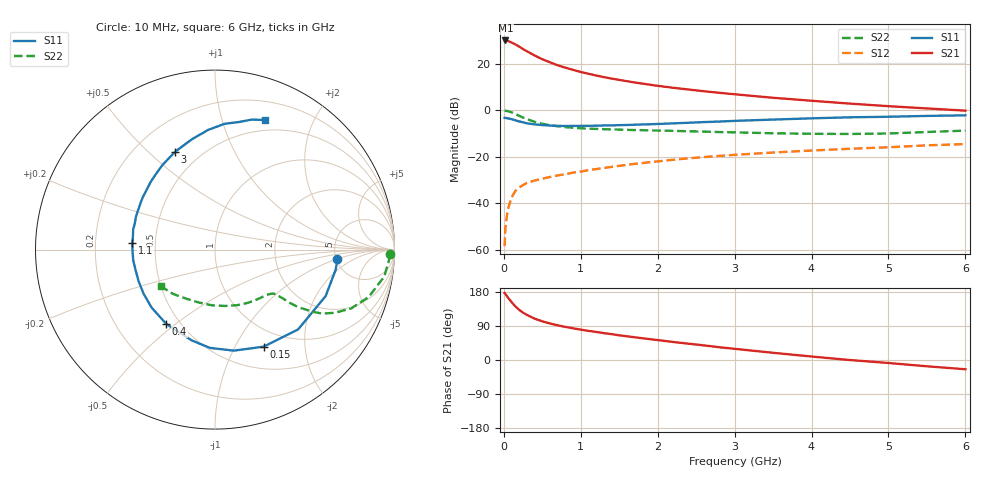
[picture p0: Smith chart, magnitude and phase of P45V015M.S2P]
! SIEMENS Small Signal Semiconductors
! BFP182
! Si NPN RF Bipolar Junction Transistor in SOT143
! VCE = 5 V  IC = 15 mA
! Common Emitter S-Parameters:  March  1996
# GHz  S  MA  R  50
!  f  S11  S21  S12  S22
! GHz  MAG  ANG  MAG  ANG  MAG  ANG  MAG  ANG
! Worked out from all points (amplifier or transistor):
!   36 points, 10 MHz to 6 GHz, reference 50 ohm
!   highest |S21| = 29.9 dB at 20 MHz (marker M1)
!   |S21| within 3 dB of that: start of sweep to 216.3 MHz
!   unconditionally stable (mu >= 1): 978.4 MHz to 5.403 GHz
!   at 250 MHz: K = 0.40, MSG = 29.2 dB, |S12| = -32.2 dB
!   at 1.4 GHz: K = 1.11, MAG = 17.0 dB, |S12| = -24.4 dB
!   at 6 GHz: K = 0.94, MSG = 7.2 dB, |S12| = -14.6 dB
!   S11 on the Smith chart (normalised r, x): 10 MHz: 5.11, -1.05; 150 MHz: 0.77, -1.31; 400 MHz: 0.42, -0.46; 1.1 GHz: 0.37, +0.03; 3 GHz: 0.36, +0.61; 6 GHz: 0.38, +1.39
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0.01  0.6841 -4.6  31.32 176.8  0.0012 91.1  0.973 -1.6
0.02  0.6817 -9.4  31.42 174.3  0.0029 82.6  0.971 -3.6
0.05  0.6687 -22.8  30.87 165.6  0.0072 81.5  0.9553 -9.0
0.1  0.642 -43.8  28.34 152.9  0.0133 68.9  0.8962 -17.1
0.15  0.6048 -63.4  25.86 141.5  0.0185 63.0  0.8274 -23.3
0.2  0.5728 -79.4  23.14 132.3  0.0219 58.2  0.7549 -27.8
0.25  0.5484 -92.9  20.49 124.9  0.0246 54.7  0.6941 -30.9
0.3  0.5224 -104.4  18.38 119.0  0.0274 52.6  0.6411 -32.6
0.4  0.4949 -123.4  14.95 109.1  0.0308 49.3  0.5614 -34.7
0.5  0.4787 -137.5  12.39 102.0  0.0338 47.8  0.5095 -35.5
0.6  0.4677 -148.4  10.66 96.4  0.0368 48.3  0.4752 -35.7
0.7  0.4604 -157.9  9.204 91.5  0.0397 48.4  0.4508 -35.9
0.9  0.4594 -172.5  7.337 83.7  0.0456 49.1  0.4187 -36.3
1.1  0.4617 175.4  6.059 76.8  0.0515 50.0  0.4013 -37.7
1.5  0.4768 157.6  4.464 65.1  0.0638 49.7  0.3823 -41.6
1.8  0.4932 146.0  3.721 57.4  0.0731 48.9  0.3718 -45.7
2.2  0.5204 133.5  3.032 47.6  0.086 46.8  0.3595 -52.2
3  0.589 112.1  2.197 29.5  0.1099 40.6  0.3337 -68.2
3.5  0.6282 101.8  1.846 19.0  0.1231 36.4  0.319 -79.9
4.5  0.7031 85.6  1.383 -0.1  0.1482 28.2  0.3081 -106.6
5.5  0.7527 74.2  1.09 -16.6  0.1756 20.5  0.3399 -133.3
6  0.7746 68.8  0.977 -24.4  0.187 15.7  0.3638 -145.9
